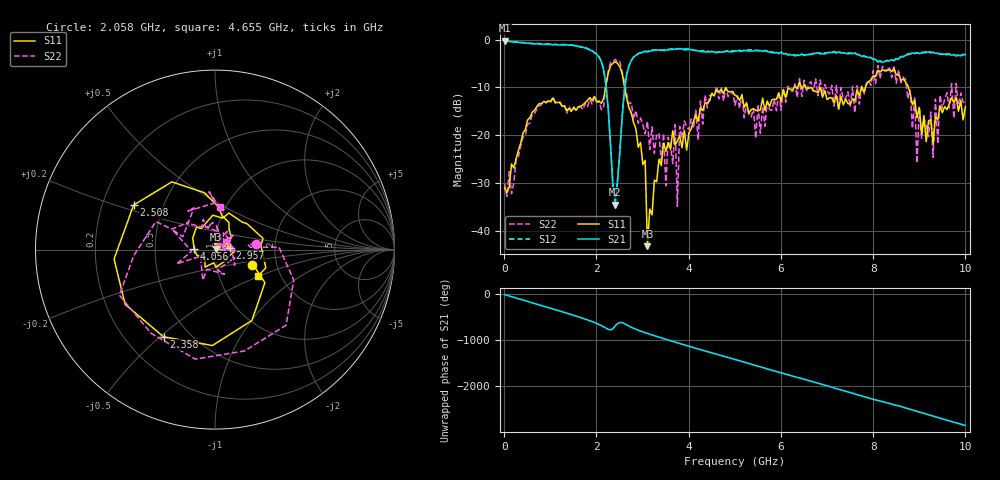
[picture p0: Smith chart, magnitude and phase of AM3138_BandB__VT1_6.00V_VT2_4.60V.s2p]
! Date/Time: Tue, Nov 13, 2018 4:40 PM
! Network Analyzer: Agilent Technologies E8364B Rev: A.07.50.67
! Sweep from 0.010 to 10.000 GHz, 201 Points, Sweep Type: LIN
! Power Supply: 6.001 V, 0.000 A
# Hz S DB R 50
!freq MagS11 AngS11 MagS21 AngS21 MagS12 AngS12 MagS22 AngS22
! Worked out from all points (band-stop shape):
!   201 points, 10 MHz to 10 GHz, reference 50 ohm
!   highest |S21| = -0.26 dB at 10 MHz (marker M1); lowest = -34.5 dB at 2.408 GHz (marker M2)
!   |S21| within 3 dB of the highest: start of sweep to 2.021 GHz; 2.862 GHz to 6.266 GHz (3.404 GHz wide, 74.6 % of centre)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
!   lowest |S11| = -43.2 dB at 3.107 GHz (marker M3), VSWR 1.01, Z = 50.5 + j0.427 ohm
!   |S11| at or under -10 dB: start of sweep to 2.199 GHz; 2.611 GHz to 6.286 GHz (3.675 GHz wide, 82.6 % of centre); 8.762 GHz to end of sweep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
!   |S22| runs from -34.9 to -4.2 dB; largest |S21 - S12| = 0.026
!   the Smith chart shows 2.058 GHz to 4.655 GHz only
!   S11 on the Smith chart (normalised r, x): 2.058 GHz: 1.50, -0.27; 2.358 GHz: 0.36, -0.51; 2.508 GHz: 0.34, +0.23; 2.957 GHz: 1.18, +0.02; 4.056 GHz: 0.79, +0.01; 4.655 GHz: 1.54, -0.49
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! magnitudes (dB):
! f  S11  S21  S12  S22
! 10 MHz  -31.0  -0.3  -0.2  -30.2
! 1.708 GHz  -13.7  -1.6  -1.6  -14.6
! 2.058 GHz  -13.0  -3.7  -3.6  -12.8
! 2.358 GHz  -5.0  -30.5  -30.5  -4.6
! 2.408 GHz  -4.6  -34.5  -34.1  -4.2
! 2.508 GHz  -5.7  -23.7  -23.5  -4.6
! 2.957 GHz  -21.6  -2.8  -2.8  -16.4
! 3.107 GHz  -43.2  -2.6  -2.5  -17.1
! 3.357 GHz  -25.1  -2.2  -2.2  -19.7
! 3.507 GHz  -23.4  -2.2  -2.1  -30.6
! 3.706 GHz  -22.1  -2.0  -1.9  -17.8
! 3.756 GHz  -21.2  -1.9  -2.0  -34.9
! 3.806 GHz  -20.2  -2.0  -1.9  -18.2
! 4.056 GHz  -18.6  -2.1  -2.1  -16.7
! 4.655 GHz  -11.0  -2.6  -2.6  -12.4
! 5.005 GHz  -11.7  -2.4  -2.4  -13.8
! 6.703 GHz  -10.7  -3.0  -2.8  -10.8
! 8.352 GHz  -6.3  -4.4  -4.5  -5.6
! 8.901 GHz  -12.7  -2.9  -2.9  -12.1
! 8.951 GHz  -16.4  -2.8  -2.7  -25.9
! 9.001 GHz  -14.2  -2.9  -2.8  -14.1
! 10 GHz  -14.0  -3.1  -3.0  -13.3
